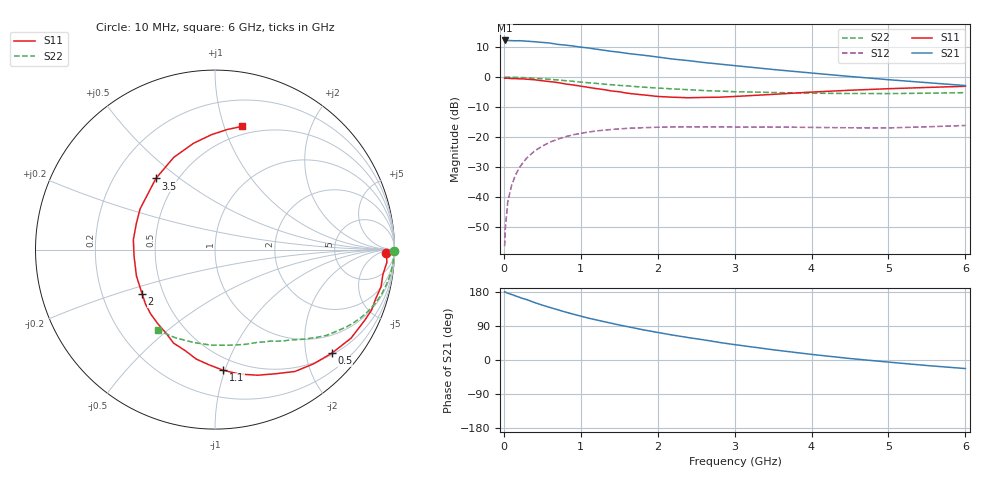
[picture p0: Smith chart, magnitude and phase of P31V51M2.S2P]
! SIEMENS Small Signal Semiconductors
! BFP181
! Si NPN RF Bipolar Junction Transistor in SOT143
! VCE = 1.5 V  IC = 1.2 mA
! Common Emitter S-Parameters:  March  1996
# GHz  S  MA  R  50
!  f  S11  S21  S12  S22
! GHz  MAG  ANG  MAG  ANG  MAG  ANG  MAG  ANG
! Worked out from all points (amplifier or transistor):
!   36 points, 10 MHz to 6 GHz, reference 50 ohm
!   highest |S21| = 12.3 dB at 10 MHz (marker M1)
!   |S21| within 3 dB of that: start of sweep to 1.228 GHz
!   unconditionally stable (mu >= 1): 2.831 GHz to end of sweep
!   at 250 MHz: K = 0.10, MSG = 20.3 dB, |S12| = -28.5 dB
!   at 1.4 GHz: K = 0.55, MSG = 13.1 dB, |S12| = -17.5 dB
!   at 6 GHz: K = 1.28, MAG = 3.5 dB, |S12| = -16.2 dB
!   S11 on the Smith chart (normalised r, x): 10 MHz: 38, -15; 500 MHz: 0.54, -2.54; 1.1 GHz: 0.40, -0.99; 2 GHz: 0.38, -0.24; 3.5 GHz: 0.38, +0.41; 6 GHz: 0.42, +1.15
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0.01  0.9553 -1.0  4.098 179.6  0.0015 82.8  0.9989 -0.3
0.02  0.956 -1.6  4.078 179.2  0.003 85.6  0.9981 -0.8
0.05  0.9603 -4.2  4.092 176.4  0.0081 89.7  0.9961 -2.0
0.1  0.9457 -8.5  4.071 172.9  0.0154 83.9  0.995 -4.0
0.15  0.9479 -12.7  4.045 169.3  0.0229 81.3  0.9911 -5.9
0.2  0.9366 -16.8  4.063 165.6  0.0305 78.9  0.9876 -7.8
0.3  0.9229 -25.2  3.982 159.2  0.0448 74.1  0.9742 -11.7
0.4  0.9043 -33.1  3.903 151.6  0.0584 68.6  0.9603 -15.3
0.5  0.8701 -41.5  3.801 144.8  0.0705 63.4  0.94 -18.8
0.6  0.841 -49.1  3.706 138.6  0.082 58.8  0.9184 -22.1
0.8  0.7696 -64.0  3.428 126.6  0.1008 50.2  0.8732 -27.8
1.1  0.6744 -86.0  3.069 110.5  0.1209 39.6  0.8048 -35.1
1.3  0.6189 -99.7  2.815 101.3  0.1301 33.4  0.7647 -39.2
1.5  0.5699 -113.9  2.609 92.4  0.1363 28.3  0.7277 -42.6
1.8  0.5068 -135.0  2.335 80.1  0.1429 22.5  0.6826 -47.2
2  0.4753 -148.7  2.165 72.7  0.1454 19.0  0.6567 -50.0
2.2  0.4616 -161.5  2.002 65.6  0.1471 15.6  0.6361 -53.1
2.8  0.4618 161.6  1.653 46.4  0.1476 8.7  0.5849 -61.6
3.5  0.5154 129.7  1.342 27.0  0.1468 3.8  0.5538 -72.5
4.5  0.604 101.5  1.026 3.9  0.1426 0.5  0.5329 -92.3
5.5  0.672 84.3  0.809 -14.6  0.1479 2.1  0.5385 -114.0
6  0.7031 77.6  0.723 -22.6  0.1557 2.2  0.5506 -125.1
